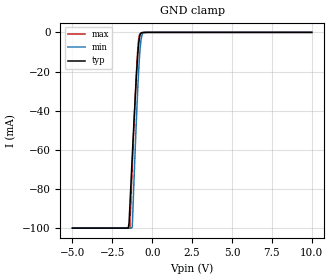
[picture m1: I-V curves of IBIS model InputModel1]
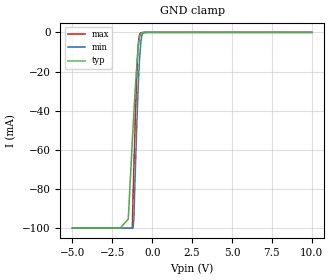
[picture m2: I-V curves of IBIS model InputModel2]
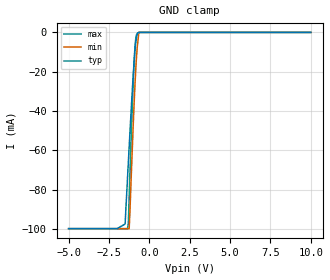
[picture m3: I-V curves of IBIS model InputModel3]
[IBIS Ver]   2.1
[File name]   pa_200bx.ibs   |pa_=PSOP, f200bx=abbr. chip name, 5=5V Vcc
[File Rev]   2.0
[Date]   14-February-1996
[Source]   File generated from lab measurements at Intel Corporation.
[Notes]   Rev 2.0 All data was replaced by actual measurements
   performed in a lab.
[Disclaimer] INTEL DEVELOPER'S SOFTWARE LICENSE AGREEMENT
| BY USING THIS SOFTWARE, YOU ARE AGREEING TO BE BOUND
| BY THE TERMS OFTHIS AGREEMENT.  DO NOT USE THE SOFTWARE
| UNTIL YOU HAVE CAREFULLY READAND AGREED TO THE FOLLOWING
| TERMS AND CONDITIONS.  IF YOU DO NOT AGREETO THE TERMS
| OF THIS AGREEMENT, PROMPTLY RETURN THE SOFTWARE PACKAGE
| ANDANY ACCOMPANYING ITEMS.
| IF YOU USE THIS SOFTWARE, YOU WILL BE BOUND BY THE TERMS
| OF THIS AGREEMENT
| LICENSE: Intel Corporation ("Intel") grants you the non-exclusive right
| to use the enclosed software program ("Software").  You will not use,
| copy, modify, rent, sell or transfer the Software or any portion
| thereof, except as provided in this Agreement.
| System OEM Developers may:
| 1.   Copy the Software for support, backup or archival purposes;
| 2.   Install, use, or distribute Intel owned Software in object code
|   only;
| 3.   Modify and/or use Software source code that Intel directly makes
|   available to you as an OEM Developer;
| 4.   Install, use, modify, distribute, and/or make or have made
|   derivatives ("Derivatives") of Intel owned Software under the
|   terms and conditions in this Agreement, ONLY if you are a System
|   OEM Developer and NOT an end-user.
| RESTRICTIONS:
| YOU WILL NOT:
| 1.   Copy the Software, in whole or in part, except as provided for
|   in this Agreement;
| 2.   Decompile or reverse engineer any Software provided in object
|   code format;
| 3.   Distribute any Software or Derivative code to any end-users,
|   unless approved by Intel in a prior writing.
| TRANSFER: You may transfer the Software to another OEM
| Developer if thereceiving party agrees to the terms of this
| Agreement at the sole risk of any receiving party.
| OWNERSHIP AND COPYRIGHT OF SOFTWARE:
| Title to the Software and all copies thereof remain with Intel
| or its vendors.  The Software iscopyrighted and is protected by
| United States and international copyright laws.  You will not
| remove the copyright notice from the Software.  You agree to
| prevent any unauthorized copying of the Software.
| DERIVATIVE WORK: OEM Developers that make or have made
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[Copyright]   Copyright 1996, Intel Corporation, All Rights Reserved
[Component]   PA28F200BX   | 44-lead PSOP package, 28F200BX
[Manufacturer]  Intel   | Boot Block(tm) Memory
|   | operating in 5V Vcc range
[Package]
|Variable   typ   min   max
R_pkg   145.5m   144.0m   147.0m
L_pkg   5.25nH   2.00nH   8.50nH
C_pkg   1.09pF   0.68pF   1.50pF
|***********************Pin Definition********************************
[Pin]   signal_name   model_name   R_pin   L_pin   C_pin
  1   VPP   POWER
  2   DU   InputModel6
  3   A17   InputModel1
  4   A7   InputModel1
  5   A6   InputModel1
  6   A5   InputModel1
  7   A4   InputModel1
  8   A3   InputModel1
  9   A2   InputModel1
 10   A1   InputModel1
 11   A0   InputModel2
 12   CE#   InputModel2
 13   GND   GND
 14   OE#   InputModel4
 15   DQ0   InputOutput1
 16   DQ8   InputOutput1
 17   DQ1   InputOutput1
 18   DQ9   InputOutput1
 19   DQ2   InputOutput1
 20   DQ10   InputOutput1
 21   DQ3   InputOutput1
 22   DQ11   InputOutput1
 23   VCC   POWER
 24   DQ4   InputOutput1
 25   DQ12   InputOutput1
 26   DQ5   InputOutput1
 27   DQ13   InputOutput1
 28   DQ6   InputOutput1
 29   DQ14   InputOutput1
 30   DQ7   InputOutput1
 31   DQ15   InputOutput2
 32   GND   GND
 33   BYTE#   InputModel2
 34   A16   InputModel2
 35   A15   InputModel1
 36   A14   InputModel1
 37   A13   InputModel1
 38   A12   InputModel1
 39   A11   InputModel1
 40   A10   InputModel1
 41   A9   InputModel1
 42   A8   InputModel1
 43   WE#   InputModel5
 44   RP#   InputModel3
|**************************Input Model 6****************************
[Model]   InputModel6
Model_type   Input
|   Model for DU & NC pins Excluding Pin #3.
Vinl = 0.8V
Vinh = 2.0V
|Variable   typ   min   max
C_comp   4.91p   NA   6.50p
[Voltage Range]   5.0V   4.5V   5.5V
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| Models and submodels in the file (8): InputModel1 (Input), InputModel2 (Input), InputModel3 (Input), InputModel4 (Input), InputModel5 (Input), InputModel6 (Input), InputOutput1 (I/O), InputOutput2 (I/O)
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|***************************Input Model 1****************************
[Model]   InputModel1
Model_type   Input
|   Model for A[15:1] & Pin 3 (NC)
Vinl = 0.8V
Vinh = 2.0V
|Variable   typ   min   max
C_comp   4.91p   NA   6.50p
[Voltage Range]   5.0V   4.5V   5.5V
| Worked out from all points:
|   GND clamp passes 1 mA (typ) near -0.75 V on its own axis
[GND_clamp]
|Voltage   I(typ)   I(min)   I(max)
-5V       -99.84mA   -99.85mA   -99.85mA
-1.5V     -99.84mA   -99.85mA   -99.85mA
-1.45V    -97.1mA    -99.85mA   -99.85mA
-1.4V     -88.66mA   -99.85mA   -99.85mA
-1.25V    -63.24mA   -99.36mA   -69.05mA
-1.05V    -31.09mA   -56.35mA   -30.63mA
-950mV    -16.83mA   -36.7mA    -14.35mA
-850mV    -5.99mA    -19.86mA   -3.6mA
-750mV    -1.015mA   -7.435mA   -471.4uA
-650mV    -202.7uA   -1.654mA   -140.8uA
-500mV    -27.26uA   -101.4uA   -12.27uA
10V       0A         0A         0A
[Power_clamp]
| Input buffer circuits of this product do not intrinisically
| require a [Power_clamp] defintion.  This zero current
| [Power_clamp] table is provided for the compatibility with
| some IBIS parsers.
|Voltage   I(typ)   I(min)   I(max)
-5V       0A         0A         0A
0V        0A         0A         0A
5V        0A         0A         0A
10V       0A         0A         0A
|***************************Input Model 2****************************
[Model]   InputModel2
Model_type   Input
|   Model for A[0], A[16], CE# & BYTE#
Vinl = 0.8V
Vinh = 2.0V
|Variable   typ   min   max
C_comp   4.91p   NA   6.50p
[Voltage Range]   5.0V   4.5V   5.5V
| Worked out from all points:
|   GND clamp passes 1 mA (typ) near -0.75 V on its own axis
[GND_clamp]
|Voltage   I(typ)   I(min)   I(max)
-5V       -99.84mA   -99.85mA   -99.85mA
-2V       -99.84mA   -99.85mA   -99.85mA
-1.5V     -95.21mA   -99.85mA   -99.85mA
-1.25V    -55.95mA   -99.85mA   -99.68mA
-1.2V     -48.44mA   -99.85mA   -84.47mA
-1.15V    -41.14mA   -95.68mA   -69.64mA
-950mV    -15.15mA   -43.95mA   -18.45mA
-850mV    -5.666mA   -23.02mA   -4.089mA
-750mV    -1.032mA   -9.168mA   -475.6uA
-650mV    -207.5uA   -1.728mA   -133.8uA
-500mV    -28.64uA   -98.99uA   -10.29uA
10V       0A         0A         0A
[Power_clamp]
| Input buffer circuits of this product do not intrinisically
| require a [Power_clamp] defintion.  This zero current
| [Power_clamp] table is provided for the compatibility with
| some IBIS parsers.
|Voltage   I(typ)   I(min)   I(max)
-5V       0A         0A         0A
0V        0A         0A         0A
5V        0A         0A         0A
10V       0A         0A         0A
|***************************Input Model 3****************************
[Model]   InputModel3
Model_type   Input
|   Model for RP#
Vinl = 0.8V
Vinh = 2.0V
|Variable   typ   min   max
C_comp   4.91p   NA   6.50p
[Voltage Range]   5.0V   4.5V   5.5V
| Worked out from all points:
|   GND clamp passes 1 mA (typ) near -0.75 V on its own axis
[GND_clamp]
|Voltage   I(typ)   I(min)   I(max)
-5V       -99.85mA   -99.85mA   -99.85mA
-2V       -99.85mA   -99.85mA   -99.85mA
-1.5V     -97.47mA   -99.85mA   -99.85mA
-1.35V    -73.75mA   -99.85mA   -99.85mA
-1.3V     -65.95mA   -99.85mA   -96.97mA
-1.25V    -58.19mA   -99.85mA   -83.97mA
-1.05V    -28.67mA   -57.7mA    -35.89mA
-950mV    -15.59mA   -37.45mA   -16.08mA
-850mV    -5.621mA   -20.13mA   -3.693mA
-750mV    -981uA     -7.476mA   -460uA
-650mV    0A         0A         0A
10V       0A         0A         0A
[Power_clamp]
| Input buffer circuits of this product do not intrinisically
| require a [Power_clamp] defintion.  This zero current
| [Power_clamp] table is provided for the compatibility with
| some IBIS parsers.
|Voltage   I(typ)   I(min)   I(max)
-5V       0A         0A         0A
0V        0A         0A         0A
5V        0A         0A         0A
10V       0A         0A         0A
